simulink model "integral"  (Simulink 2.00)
settings: Solver=ode45  StartTime=0.0  StopTime=10  RelTol=1e-3  AbsTol=1e-6

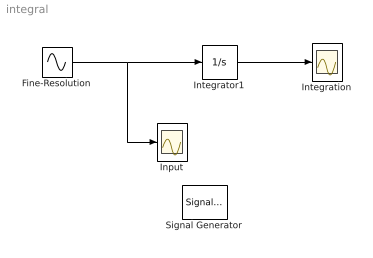
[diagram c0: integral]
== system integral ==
  Fine-Resolution : Sin  Amplitude=1  Frequency=4  Phase=0  SampleTime=0.01
  Input : Scope
  Integration : Scope
  Integrator1 : Integrator  ExternalReset=none  InitialConditionSource=internal  InitialCondition=-0.25  LimitOutput=off  UpperSaturationLimit=inf  LowerSaturationLimit=-inf  ShowSaturationPort=off  ShowStatePort=off  AbsoluteTolerance=auto
  Signal Generator : SignalGenerator  WaveForm=sine  Amplitude=1  Frequency=8  Units=rad/sec
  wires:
  Fine-Resolution/1 -> Input/1, Integrator1/1
  Integrator1/1 -> Integration/1
